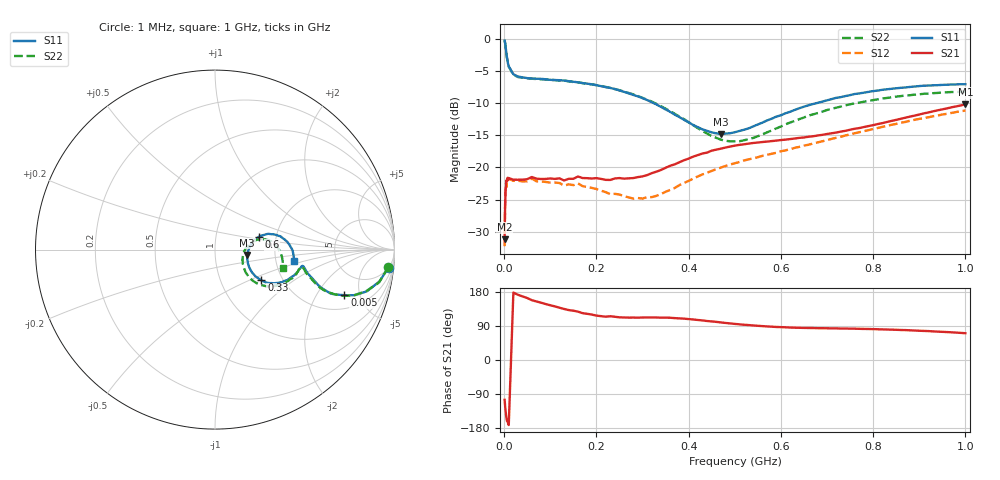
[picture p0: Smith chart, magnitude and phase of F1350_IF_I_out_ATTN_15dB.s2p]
! S-parameters for IF_I+ & IF_I- IDT F1350 DPD Demodulator
! Date Measured:  2015-11-25  RGG
!  Port 1 = Pin 19 = IF_I+
!  Port 2 = Pin 20 = IF_I-
! State: 15 dB attenuation (Gain = Gmax - 15 dB)
! IF Frequency:  1 MHz to 1000 MHz
! RF_INX, RF_INY, IF_Q+, and IF_Q- terminated
! 2300 MHz, 0 dBm signal applied to LO_IN
! Vcc = +5.00 Volts  Icc = approx 275 mA.
! NOTES:  The device was measured on a custom printed circuit evaluation board with individual 50 ohm
!  microstrip lines to the RF and LO pins. The IF outputs are normally connected to balun
!  transformers, which convert the balanced IF output signals to single ended (SE) 50 ohm signals
!  for normal test purposes. For these measurements, to measure the IFI+ and IFI- output SE s-parameters,
!  the chokes associated with the IFI+ and IFI- outputs were removed and a pair of pigtailed
!  50 ohm coaxial lines were soldered to the PCB at these points. 5.00 volt bias was provided
!  to these pins via external bias tees. Data was collected using a calibrated vector
!  network analyzer.  The pigtailed 50 ohm coaxial lines were de-embedded using reference
!  plane extensions. 100 ohm microstrip lines of length 386 mils and 218 mils for the IF_I+ and IF_I-
!  signals, respectively, were de-embedded using Agilent ADS, yielding the reference plane at the IC edge.
!  Only IFI+ and IFI- outputs were measured. IF_Q+ and IF_Q- should be identical.
!  This data is single-ended relative to ports IF_I+ and IF_I- (reference impedance = 50 ohms)
!  Common mode or differential S-parameters may be extracted from this data with a linear simulator.
# mhz S db R 50
! freq  dbS11  angS11  dbS21  angS21  dbS12  angS12  dbS22  angS22
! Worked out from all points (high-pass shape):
!   109 points, 1 MHz to 1 GHz, reference 50 ohm
!   highest |S21| = -10.20 dB at 1 GHz (marker M1); lowest = -31.2 dB at 1 MHz (marker M2)
!   |S21| within 3 dB of the highest: 813.2 MHz to end of sweep
!   lowest |S11| = -14.8 dB at 470 MHz (marker M3), VSWR 1.45, Z = 71.8 - j4.38 ohm
!   |S11| at or under -10 dB: 324.4 MHz to 676.9 MHz (352.5 MHz wide, 70.4 % of centre)
!   |S22| runs from -15.9 to -0.3 dB; largest |S21 - S12| = 0.066
!   S11 on the Smith chart (normalised r, x): 1 MHz: 5, -18; 5 MHz: 2.92, -3.57; 330 MHz: 1.56, -0.59; 600 MHz: 1.62, +0.25; 1 GHz: 2.52, -0.40
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1  -0.25 -5.9  -31.17 -104.9  -32.23 -107.6  -0.26 -5.8
2  -0.61 -11.0  -26.41 -120.3  -25.94 -120.9  -0.61 -11.3
3  -1.14 -15.4  -23.69 -132.9  -23.59 -133.9  -1.18 -15.4
4  -1.72 -18.0  -22.99 -144.0  -22.43 -143.5  -1.76 -18.1
5  -2.33 -19.4  -21.99 -152.7  -23.05 -149.7  -2.35 -19.8
6  -2.82 -20.3  -22.13 -160.5  -22.10 -158.1  -2.93 -20.5
10  -4.28 -19.1  -21.65 -171.7  -21.74 -171.0  -4.32 -19.5
20  -5.50 -14.2  -21.90 178.0  -22.08 178.5  -5.58 -14.5
60  -6.16 -10.8  -21.48 157.9  -21.70 159.2  -6.20 -11.3
130  -6.49 -15.9  -22.02 134.7  -22.83 136.8  -6.48 -16.7
160  -6.76 -18.8  -21.40 127.6  -22.48 129.2  -6.75 -20.3
170  -6.88 -19.6  -21.64 123.6  -22.90 125.7  -6.88 -21.0
280  -8.71 -30.6  -21.64 112.0  -24.84 115.3  -8.63 -33.6
330  -10.19 -33.4  -20.65 112.2  -24.42 121.9  -10.11 -38.3
340  -10.57 -33.6  -20.38 111.7  -24.13 123.5  -10.46 -38.9
430  -14.07 -22.2  -17.82 104.4  -21.08 122.9  -14.32 -32.7
470  -14.78 -9.3  -17.07 99.1  -20.02 119.5  -15.68 -21.3
510  -14.32 3.1  -16.48 94.1  -19.15 115.9  -15.92 -7.7
600  -11.88 16.2  -15.73 86.7  -17.48 109.0  -13.63 11.2
670  -10.12 16.4  -15.14 84.3  -16.26 105.0  -11.74 12.9
840  -7.76 5.2  -12.76 80.0  -13.36 92.5  -9.09 1.2
1000  -7.05 -8.2  -10.20 70.6  -11.14 78.4  -8.19 -15.0
